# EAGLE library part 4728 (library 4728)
Adafruit Accessories Replacement CSI/DSI Connector for Raspberry Pi - Repair Part Source: Datasheet
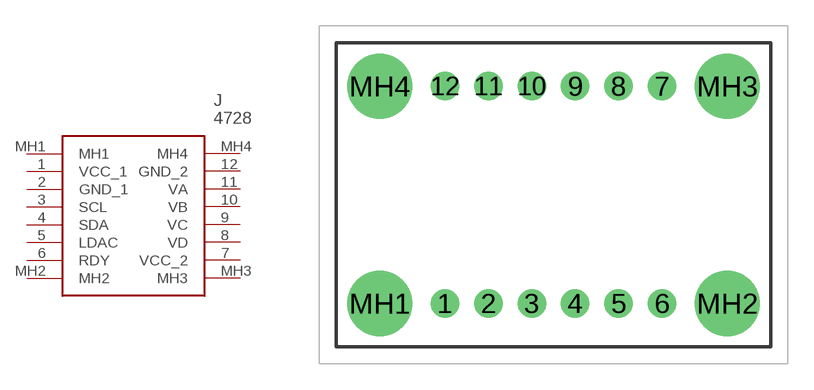
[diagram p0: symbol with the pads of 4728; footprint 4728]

Designator prefix J

## 4728 (Description: Adafruit Accessories Replacement CSI/DSI Connector for Raspberry Pi - Repair Part; Height: 4.6mm; Manufacturer_Name: Adafruit; Manufacturer_Part_Number: 4728; Mouser_Part_Number: 485-4728; Mouser_Price-Stock: https://www.mouser.co.uk/ProductDetail/Adafruit/4728?qs=hd1VzrDQEGjMsIeQ7t%2FzlA%3D%3D)  [4728]
1  VCC_1
2  GND_1
3  SCL
4  SDA
5  LDAC
6  RDY
7  VCC_2
8  VD
9  VC
10  VB
11  VA
12  GND_2
MH1  MH1
MH2  MH2
MH3  MH3
MH4  MH4

## Footprint 4728 (pad centres in mm)
4728-2
drill 1.11 pad 1.665: 1 0,0; 2 2.54,0; 3 5.08,0; 4 7.62,0; 5 10.16,0; 6 12.7,0; 7 12.7,12.7; 8 10.16,12.7; 9 7.62,12.7; 10 5.08,12.7; 11 2.54,12.7; 12 0,12.7
drill 2.54 pad 3.81: MH1 -3.81,0; MH2 16.51,0; MH3 16.51,12.7; MH4 -3.81,12.7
